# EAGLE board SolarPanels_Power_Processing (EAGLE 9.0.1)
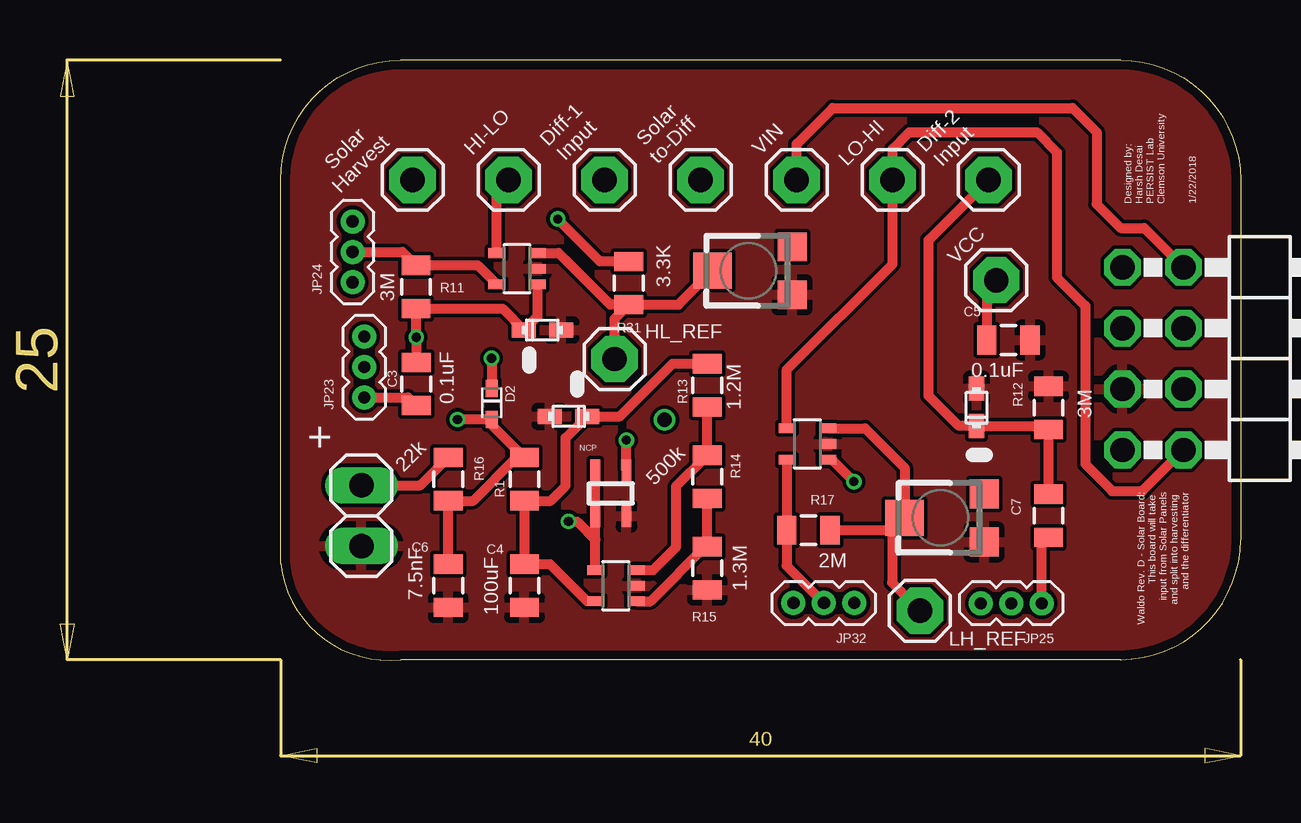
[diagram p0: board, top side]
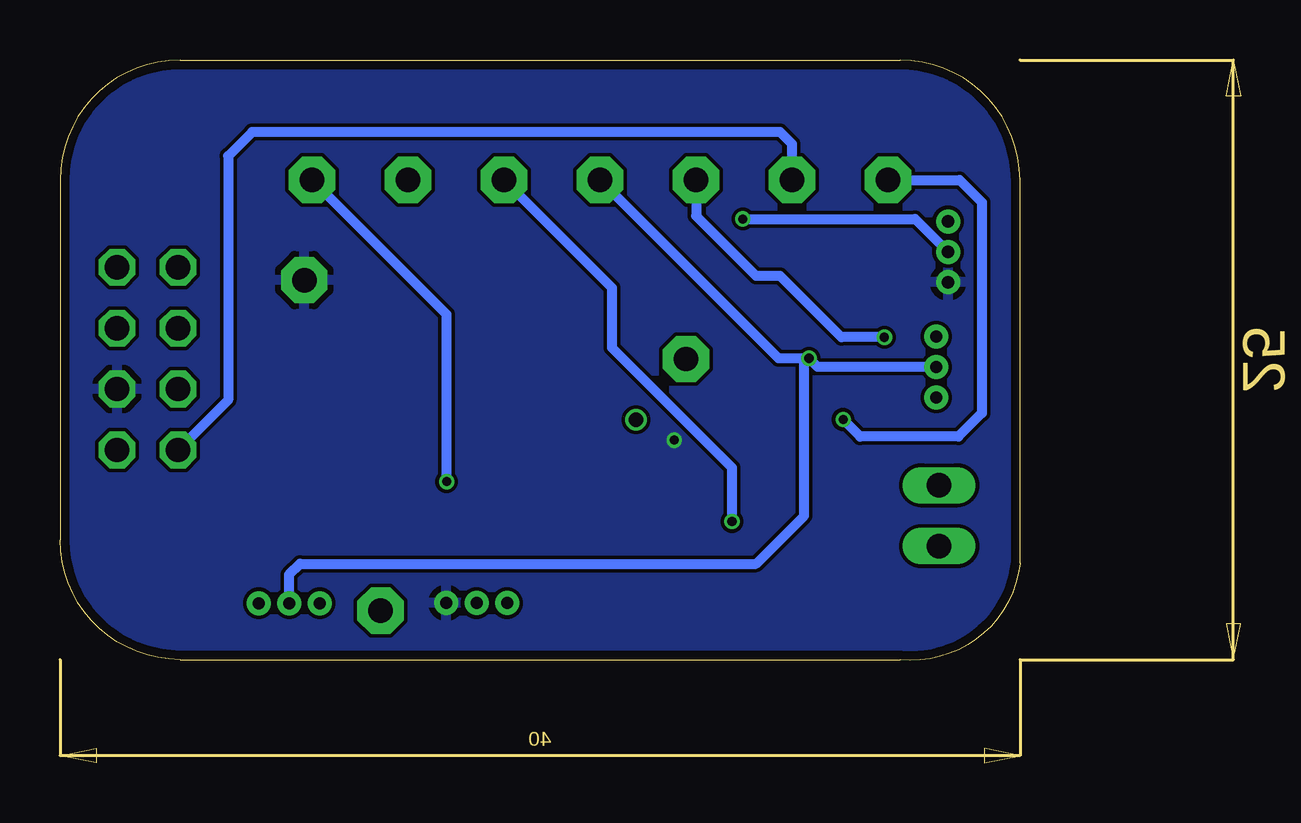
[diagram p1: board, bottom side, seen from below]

Size 49.19 x 29.3 mm. Coordinates in mm from the lower left corner, seen from the top.
Outline: 44.19,29.3 14.19,29.3 arc90 9.19,24.3 9.19,8.31 arc90 14.19,4.3 44.19,4.3 arc90 49.19,9.3 49.19,24.3 arc90 44.19,29.3
Copper layers (1*16): Top 0.035559375mm / dielectric 1.6mm / Bottom 0.035559375mm
Design rules "oshpark-2layer": minimum track width 6mil, minimum drill 10mil, track to track 6mil, track to pad 6mil, pad to pad 6mil, via to via 6mil, smd to smd 6mil, copper to edge 15mil, drill to drill 6mil, minimum pad ring 5mil, minimum via ring 5mil, stop-mask expansion 2.5mil, vias tented up to drill 0mil, thermal gap 10mil

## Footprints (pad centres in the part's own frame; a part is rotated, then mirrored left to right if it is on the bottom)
0805 = smd 0.8 x 1.2: 1 -0.9,0; 2 0.9,0
SOD523 = smd 0.7 x 0.5: A 0.7,0; C -0.6,0
1X01 = drill 1.016 pad 1.93 octagon: 1 0,0
SC70-5 = smd 0.4 x 0.7: 1 -0.65,-0.85; 2 0,-0.85; 3 0.65,-0.85; 4 0.65,0.85; 5 -0.65,0.85
2X04/90 = drill 1.016 octagon: 1 -3.81,-6.35; 2 -3.81,-3.81; 3 -1.27,-6.35; 4 -1.27,-3.81; 5 1.27,-6.35; 6 1.27,-3.81; 7 3.81,-6.35; 8 3.81,-3.81
1X03-1.27MM = drill 0.508 pad 1: 1 -1.27,0; 2 0,0; 3 1.27,0
SC82-AB_1PRIMARY = smd 0.406 x 0.914: 1 -1.321,-0.813; 2 -0.025,-0.813; 3 -0.025,1.067; 4 -1.321,1.067
1X02 = drill 1.016 long: 1 -1.27,0; 2 1.27,0
TC33X = smd 1.2 x 1.2: 1 -1,-1.825; 3 1,-1.825 | smd 1.5 x 1.6: 2 0,1.5
SOD-523 = smd 1 x 0.635: ANODE -0.8,0; CATHODE 0.76,0

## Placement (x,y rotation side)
3.3K  R31  [0805]  23.7,20 270 top
C3  0.1uF  [0805]  14.85,15.79 90 top
C4  100uF  [0805]  19.35,7.38 90 top
C5  0.1uF  [0805]  39.52,17.62 0 top
C6  7.5nF  [0805]  16.18,7.38 90 top
C7  0.1uF  [0805]  41.19,10.3 90 top
D2  [SOD523]  18,15 270 top
DIFF-INP-1  [1X01]  22.69,24.3 0 top
DIFF_IN2  [1X01]  38.69,24.3 0 top
HI-LO  [1X01]  18.69,24.3 0 top
HI-LO-3  TLV3691  [SC70-5]  19.04,20.6 90 top
HL_REF  [1X01]  23.11,16.83 0 top
JP1  [2X04/90]  50.62,16.85 270 top
JP23  [1X03-1.27MM]  12.68,16.5 90 top
JP24  [1X03-1.27MM]  12.19,21.3 90 top
JP25  [1X03-1.27MM]  39.64,6.65 180 top
JP32  [1X03-1.27MM]  31.83,6.66 180 top
LH_REF  [1X01]  35.83,6.34 0 top
LO-HI  [1X01]  34.69,24.3 0 top
LO-HI-3  TLV3691  [SC70-5]  31.14,13.29 90 top
MIC  MIC841  [SC70-5]  23.16,7.38 90 top
NCP  NCP583  [SC82-AB_1PRIMARY]  23.62,11.11 0 top
R1  [0805]  19.35,11.82 90 top
R11  3M  [0805]  14.84,19.84 90 top
R12  3M  [0805]  41.19,14.8 90 top
R13  1.2M  [0805]  26.97,15.73 90 top
R14  500k  [0805]  26.97,11.92 90 top
R15  1.3M  [0805]  26.97,8.11 90 top
R16  22k  [0805]  16.18,11.82 270 top
R17  2M  [0805]  31.18,9.7 0 top
SOLAR3  [1X02]  12.56,10.3 90 top
SOLAR-DIFF  [1X01]  26.69,24.3 0 top
SOLAR-HARV  [1X01]  14.69,24.3 0 top
TM1  [TC33X]  28.68,20.51 90 top
TM2  [TC33X]  36.68,10.21 90 top
VCC  [1X01]  39.01,20.12 0 top
VIN  [1X01]  30.69,24.3 0 top
ZENER1  RB751  [SOD-523]  20.09,18.04 180 top
ZENER2  RB751  [SOD-523]  21.2,14.44 0 top
ZENER3  RB751  [SOD-523]  38.19,14.8 270 top

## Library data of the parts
3.3K R1 R11-R17 = SparkFun-Resistors
C3-C7 = SparkFun-Capacitors
D2 = SparkFun-DiscreteSemi
DIFF-INP-1 DIFF_IN2 HI-LO HL_REF LH_REF LO-HI SOLAR-DIFF SOLAR-HARV TM1 TM2 VCC VIN = adafruit
HI-LO-3 LO-HI-3 = fedpower
JP1 SOLAR3 = pinhead
JP23-JP25 JP32 = SparkFun-Connectors
MIC = mic841
NCP = ncp583
ZENER1-ZENER3 = Parts

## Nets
DIFF_IN1: C3.2 DIFF-INP-1.1 HI-LO-3.1 R11.1 ZENER1.CATHODE
DIFF_IN2: C7.2 DIFF_IN2.1 LO-HI-3.1 R12.1 ZENER3.CATHODE
DIFF_POT_3: 3.3K.2 HI-LO-3.3 HL_REF.1 TM1.2
DIFF_POT_4: LH_REF.1 LO-HI-3.3 R17.2 TM2.2
DIFF_PWR1: 3.3K.1 HI-LO-3.5 JP24.2 R11.2
DIFF_PWR2: JP32.2 LO-HI-3.5 R17.1
GND: C4.1 C5.2 C6.1 HI-LO-3.2 JP1.5 LO-HI-3.2 MIC.2 NCP.2 R12.2 R15.1 SOLAR3.1 TM1.1 TM2.1 ZENER1.ANODE ZENER2.ANODE ZENER3.ANODE
HI-LO-DIFF-2: HI-LO-3.4 HI-LO.1 JP1.7
LO-HI-DIFF-2: JP1.8 LO-HI-3.4 LO-HI.1
MIC_INPUT: C4.2 MIC.5 R1.1 R13.2 ZENER2.CATHODE
N$11: MIC.3 R13.1 R14.2
N$12: MIC.1 R14.1 R15.2
SOLAR1: R16.1 SOLAR3.2
SOLAR1-1: C3.1 JP23.1
SOLAR1-2: C7.1 JP25.1
SOLAR_DIFF: D2.C JP23.2 JP25.2 SOLAR-DIFF.1
SOLAR_HARVEST: C6.2 D2.A R1.2 R16.2 SOLAR-HARV.1
VCC: C5.1 JP1.6 JP24.1 JP32.1 NCP.3 VCC.1
VIN: JP1.2 MIC.4 NCP.1 NCP.4 VIN.1
WP-CTRL: JP1.4

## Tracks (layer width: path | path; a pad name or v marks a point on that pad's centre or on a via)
DIFF_IN1  (via drill 0.38)
  Top 0.406: HI-LO-3.1 19.89,18.6 ZENER1.CATHODE 18.44,18.93 14.85,18.93 R11.1 v14.84,17.74 C3.2
  Bottom 0.406: v14.84,17.74 16.63,17.74 19.19,20.3 20.19,20.3 22.69,22.8 DIFF-INP-1.1
DIFF_IN2  (via drill 0.38)
  Top 0.406: C7.2 R12.1 41.05,14.04 ZENER3.CATHODE 37.45,14.04 36.19,15.3 36.19,21.8 DIFF_IN2.1 | LO-HI-3.1 32.16,12.64 v33.08,11.72
  Bottom 0.406: v33.08,11.72 33.08,18.69 DIFF_IN2.1
DIFF_POT_3
  Top 0.406: HI-LO-3.3 20.78,21.25 22.93,19.1 3.3K.2 | 3.3K.2 25.77,19.1 TM1.2 | HL_REF.1 23.11,18.51 3.3K.2
DIFF_POT_4
  Top 0.406: R17.2 34.67,9.7 | 34.67,9.7 TM2.2 35.19,12.3 33.55,13.94 LO-HI-3.3 | 34.67,9.7 34.67,7.5 LH_REF.1
DIFF_PWR1  (via drill 0.38)
  Top 0.406: JP24.2 14.28,21.3 R11.2 17.4,20.74 HI-LO-3.5 | 3.3K.1 22.51,20.9 v20.74,22.67
  Bottom 0.406: v20.74,22.67 13.56,22.67 JP24.2
DIFF_PWR2
  Top 0.406: JP32.2 30.28,8.21 R17.1 LO-HI-3.5
GND
  pour Top: 6.65,39.86 6.65,1.76 71.42,1.76 71.42,41.13 6.65,41.13
HI-LO-DIFF-2
  Top 0.406: HI-LO-3.4 18.19,23.8 HI-LO.1
  Bottom 0.406: HI-LO.1 18.69,25.8 19.19,26.3 41.19,26.3 42.19,25.3 42.19,15.12 JP1.7
LO-HI-DIFF-2
  Top 0.406: LO-HI-3.4 30.29,16.4 34.69,20.8 LO-HI.1 34.69,25.59 35.38,26.28 40.71,26.28 41.54,25.45 41.54,20.23 42.72,19.05 42.72,12.45 43.84,11.33 45.1,11.33 JP1.8
MIC_INPUT
  Top 0.406: MIC.5 21.96,6.73 20.41,8.28 C4.2 R1.1 20.45,10.93 21.07,11.55 21.07,13.55 ZENER2.CATHODE 23.33,14.44 25.52,16.63 R13.2
N$1  (via drill 0.6)
  other vias: 25.19,14.3
N$11
  Top 0.406: R13.1 R14.2 25.66,11.51 25.66,8.98 24.71,8.03 MIC.3
N$12
  Top 0.406: MIC.1 24.61,6.73 26.89,9.01 R15.2 R14.1
SOLAR1
  Top 0.406: SOLAR3.2 15.02,11.57 R16.1
SOLAR1-1
  Top 0.406: JP23.1 14.51,15.23 C3.1
SOLAR1-2
  Top 0.406: JP25.1 40.91,9.12 C7.1
SOLAR_DIFF  (via drill 0.38)
  Top 0.406: v17.98,16.86 17.98,15.62 D2.C
  Bottom 0.406: JP23.2 17.62,16.5 v17.98,16.86 | v17.98,16.86 19.25,16.86 SOLAR-DIFF.1 | JP25.2 39.64,7.85 39.19,8.3 20.19,8.3 18.19,10.3 18.19,16.65 v17.98,16.86
SOLAR_HARVEST  (via drill 0.38)
  Top 0.406: C6.2 R16.2 17.22,10.93 19.02,12.73 R1.2 18,14.08 D2.A v16.57,14.3 v16.56,14.31
  Bottom 0.406: SOLAR-HARV.1 11.71,24.3 10.78,23.37 10.78,14.58 11.76,13.6 15.85,13.6 v16.56,14.31
VCC  (via drill 0.38)
  Top 0.406: NCP.3 v23.6,13.45 | v23.6,13.45 | VCC.1 38.62,19.73 C5.1
  pour Bottom: 4.11,43.67 4.11,-0.78 73.96,-0.78 73.96,43.67
VIN  (via drill 0.38)
  Top 0.406: 22.31,9.3 NCP.1 | NCP.1 NCP.4 | MIC.4 22.31,9.3 | NCP.1 22.31,10.51 | v21.19,10.06 21.55,10.06 22.31,9.3 | VIN.1 30.69,25.8 32.19,27.3 42.19,27.3 43.19,26.3 43.19,23.3 44.19,22.3 45.17,22.3 JP1.2
  Bottom 0.406: v21.19,10.06 21.19,12.3 26.19,17.3 26.19,19.8 VIN.1

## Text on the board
tPlace: Diff-1 / Input | Solar / to-Diff | Diff-2 / Input | Solar / Harvest | Designed by: / Harsh Desai / PERSIST Lab / Clemson University | 1/22/2018 | + | Waldo Rev. D - Solar Board: / This board will take / input from Solar Panels / and split into harvesting / and the differentiator

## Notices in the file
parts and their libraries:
SparkFun-Resistors: Licensing: Creative Commons ShareAlike 4.0 International - https://creativecommons.org/licenses/by-sa/4.0
